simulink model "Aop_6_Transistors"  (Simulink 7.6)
settings: Solver=ode15s  StartTime=0.0  StopTime=10.0  RelTol=1e-3
libraries: fl_lib x20, elec_lib x8, nesl_utility x3

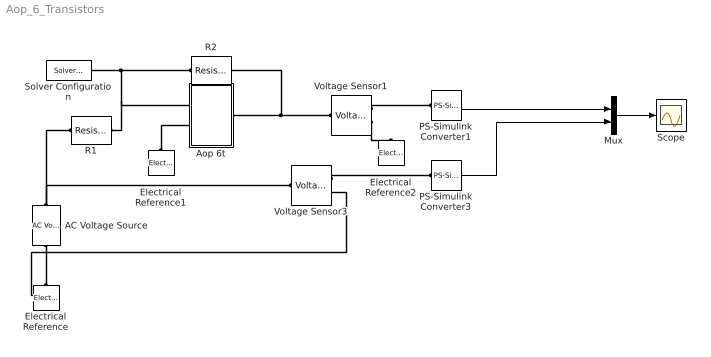
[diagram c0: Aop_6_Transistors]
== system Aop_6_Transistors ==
  AC Voltage Source : fl_lib/Electrical/Electrical Sources/AC Voltage Source  DialogController=NetworkEngine.DynNeDlgSource  SystemSampleTime=-1  amp=1 V  shift=0 rad  omega=1 Hz  i_Log=off  v_Log=off  LocalVarNames=|current|voltage|power  LocalVarDescs=|Current (A)|Voltage (V)|Power (W)  LocalVarLogging=[0 0 0]
  Aop 6t : Subsystem
  Electrical Reference : fl_lib/Electrical/Electrical Elements/Electrical Reference  DialogController=NetworkEngine.DynNeDlgSource  SystemSampleTime=-1  i_Log=off  LocalVarNames=|i  LocalVarDescs=|i  LocalVarLogging=[]
  Electrical Reference1 : fl_lib/Electrical/Electrical Elements/Electrical Reference  DialogController=NetworkEngine.DynNeDlgSource  SystemSampleTime=-1  i_Log=off  LocalVarNames=|i  LocalVarDescs=|i  LocalVarLogging=[]
  Electrical Reference2 : fl_lib/Electrical/Electrical Elements/Electrical Reference  DialogController=NetworkEngine.DynNeDlgSource  SystemSampleTime=-1  i_Log=off  LocalVarNames=|i  LocalVarDescs=|i  LocalVarLogging=[]
  Mux : Mux  Inputs=2
  PS-Simulink Converter1 : nesl_utility/PS-Simulink Converter  DialogController=NetworkEngine.DynNeUtilDlgSource  SystemSampleTime=-1  PhysicalDomain=network_engine_domain  LeftPortType=input  RightPortType=output  SubClassName=ps_output  Unit=1  AffineConversion=off
  PS-Simulink Converter3 : nesl_utility/PS-Simulink Converter  DialogController=NetworkEngine.DynNeUtilDlgSource  SystemSampleTime=-1  PhysicalDomain=network_engine_domain  LeftPortType=input  RightPortType=output  SubClassName=ps_output  Unit=1  AffineConversion=off
  R1 : fl_lib/Electrical/Electrical Elements/Resistor  DialogController=NetworkEngine.DynNeDlgSource  SystemSampleTime=-1  R=5 kOhm  i_Log=off  v_Log=off  LocalVarNames=|current|voltage|power  LocalVarDescs=|Resistor current (A)|Voltage across resistor (V)|Power (W)  LocalVarLogging=[0 0 0]
  R2 : fl_lib/Electrical/Electrical Elements/Resistor  DialogController=NetworkEngine.DynNeDlgSource  SystemSampleTime=-1  R=10 kOhm  i_Log=off  v_Log=off  LocalVarNames=|current|voltage|power  LocalVarDescs=|Resistor current (A)|Voltage across resistor (V)|Power (W)  LocalVarLogging=[0 0 0]
  Scope : Scope
  Solver Configuration : nesl_utility/Solver Configuration  DialogController=NetworkEngine.DynNeUtilDlgSource  SystemSampleTime=-1  PhysicalDomain=network_engine_domain  LeftPortType=input  RightPortType=generic  SubClassName=solver  Accelerate=off  Profile=off  ResidualTolerance=1e-9  MaxNonlinIter=12  MaxModeIter=2  DoFixedCost=off  UseLocalSampling=off  DoDC=off  LinearAlgebra=Sparse  LocalSolverSampleTime=.001  LocalSolverChoice=NE_BACKWARD_EULER_ADVANCER  UseLocalSolver=off
  Voltage Sensor1 : fl_lib/Electrical/Electrical Sensors/Voltage Sensor  DialogController=NetworkEngine.DynNeDlgSource  SystemSampleTime=-1  i1_Log=off  v1_Log=off  LocalVarNames=|i1|v1  LocalVarDescs=|i1|v1  LocalVarLogging=[]
  Voltage Sensor3 : fl_lib/Electrical/Electrical Sensors/Voltage Sensor  DialogController=NetworkEngine.DynNeDlgSource  SystemSampleTime=-1  i1_Log=off  v1_Log=off  LocalVarNames=|i1|v1  LocalVarDescs=|i1|v1  LocalVarLogging=[]
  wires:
  PS-Simulink Converter1/1 -> Mux/1
  Mux/1 -> Scope/1
  PS-Simulink Converter3/1 -> Mux/2
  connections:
  Electrical Reference/LConn1 -- Voltage Sensor3/RConn2 -- AC Voltage Source/RConn1
  AC Voltage Source/LConn1 -- Voltage Sensor3/LConn1 -- R1/LConn1
  Aop 6t/RConn1 -- R2/RConn1 -- Voltage Sensor1/LConn1
  R1/RConn1 -- Solver Configuration/RConn1 -- R2/LConn1 -- Aop 6t/LConn1
  Voltage Sensor3/RConn1 -- PS-Simulink Converter3/LConn1
  Voltage Sensor1/RConn2 -- Electrical Reference2/LConn1
  Voltage Sensor1/RConn1 -- PS-Simulink Converter1/LConn1
  Electrical Reference1/LConn1 -- Aop 6t/LConn2

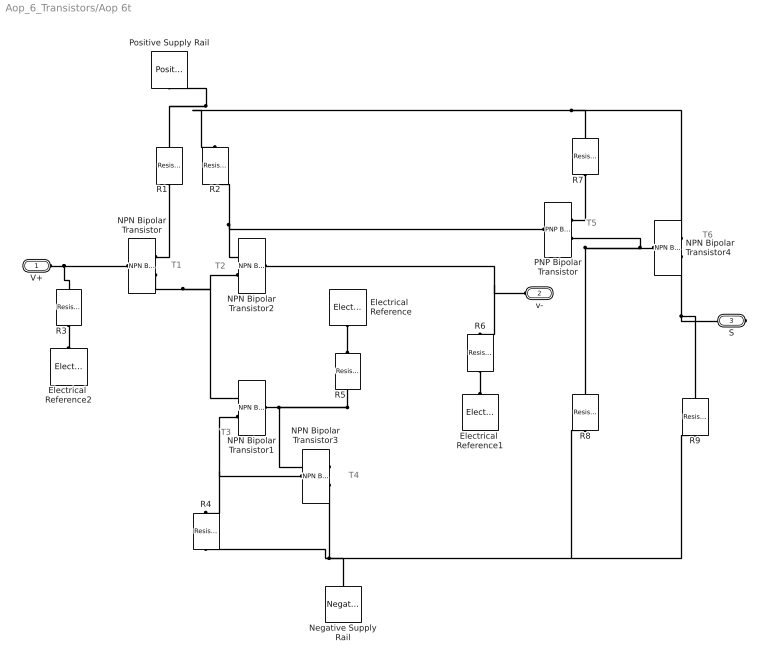
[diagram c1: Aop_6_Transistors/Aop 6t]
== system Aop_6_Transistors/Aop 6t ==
  note: T1
  note: T2
  note: T3
  note: T4
  note: T5
  note: T6
  Electrical  Reference : fl_lib/Electrical/Electrical Elements/Electrical Reference  DialogController=NetworkEngine.DynNeDlgSource  SystemSampleTime=-1  i_Log=off  LocalVarNames=|i  LocalVarDescs=|i  LocalVarLogging=0
  Electrical  Reference1 : fl_lib/Electrical/Electrical Elements/Electrical Reference  DialogController=NetworkEngine.DynNeDlgSource  SystemSampleTime=-1  i_Log=off  LocalVarNames=|i  LocalVarDescs=|i  LocalVarLogging=0
  Electrical  Reference2 : fl_lib/Electrical/Electrical Elements/Electrical Reference  DialogController=NetworkEngine.DynNeDlgSource  SystemSampleTime=-1  i_Log=off  LocalVarNames=|i  LocalVarDescs=|i  LocalVarLogging=0
  NPN Bipolar Transistor{,1..4} (5 alike) : elec_lib/Semiconductor Devices/NPN Bipolar Transistor  DialogController=NetworkEngine.DynNeDlgSource  SystemSampleTime=-1  parameterization=1  BF=100  IS=1e-14 A  VAF=200 V  hfe=100  hoe=5e-5 1/Ohm  Ic_h=1 mA  V1=0.55 V  I1=0.5 mA  BR=1  Tmeas=25 C  RC=0.01 Ohm  RE=1e-4 Ohm  RB=1 Ohm  C_BC=5 pF  C_BE=5 pF  TF=0 us  TR=0 us  LocalVarLogging=[]
  Negative Supply Rail : elec_lib/Sources/Negative Supply Rail  DialogController=NetworkEngine.DynNeDlgSource  SystemSampleTime=-1  v0=-15 V  current_Log=off  voltage_Log=off  power_Log=off  LocalVarNames=|current|voltage|power  LocalVarDescs=|Current (A)|Voltage (V)|Power (W)  LocalVarLogging=[0 0 0]
  PNP Bipolar Transistor : elec_lib/Semiconductor Devices/PNP Bipolar Transistor  DialogController=NetworkEngine.DynNeDlgSource  SystemSampleTime=-1  parameterization=1  BF=100  IS=1e-14 A  VAF=200 V  hfe=100  hoe=5e-5 1/Ohm  Ic_h=1 mA  V1=0.55 V  I1=0.5 mA  BR=1  Tmeas=25 C  RC=0.01 Ohm  RE=1e-4 Ohm  RB=1 Ohm  C_BC=5 pF  C_BE=5 pF  TF=0 us  TR=0 us  LocalVarLogging=[]
  Positive Supply Rail : elec_lib/Sources/Positive Supply Rail  DialogController=NetworkEngine.DynNeDlgSource  SystemSampleTime=-1  v0=15 V  current_Log=off  voltage_Log=off  power_Log=off  LocalVarNames=|current|voltage|power  LocalVarDescs=|Current (A)|Voltage (V)|Power (W)  LocalVarLogging=[0 0 0]
  R{1..3,6} (4 alike) : fl_lib/Electrical/Electrical Elements/Resistor  DialogController=NetworkEngine.DynNeDlgSource  SystemSampleTime=-1  R=4700 Ohm  i_Log=off  v_Log=off  LocalVarNames=|i|v  LocalVarDescs=|i|v  LocalVarLogging=[0 0]
  R4 : fl_lib/Electrical/Electrical Elements/Resistor  DialogController=NetworkEngine.DynNeDlgSource  SystemSampleTime=-1  R=1200 Ohm  i_Log=off  v_Log=off  LocalVarNames=|i|v  LocalVarDescs=|i|v  LocalVarLogging=[0 0]
  R5 : fl_lib/Electrical/Electrical Elements/Resistor  DialogController=NetworkEngine.DynNeDlgSource  SystemSampleTime=-1  R=27 kOhm  i_Log=off  v_Log=off  LocalVarNames=|i|v  LocalVarDescs=|i|v  LocalVarLogging=[0 0]
  R7 : fl_lib/Electrical/Electrical Elements/Resistor  DialogController=NetworkEngine.DynNeDlgSource  SystemSampleTime=-1  R=1 kOhm  i_Log=off  v_Log=off  LocalVarNames=|i|v  LocalVarDescs=|i|v  LocalVarLogging=[0 0]
  R8 : fl_lib/Electrical/Electrical Elements/Resistor  DialogController=NetworkEngine.DynNeDlgSource  SystemSampleTime=-1  R=24 kOhm  i_Log=off  v_Log=off  LocalVarNames=|i|v  LocalVarDescs=|i|v  LocalVarLogging=[0 0]
  R9 : fl_lib/Electrical/Electrical Elements/Resistor  DialogController=NetworkEngine.DynNeDlgSource  SystemSampleTime=-1  R=3 kOhm  i_Log=off  v_Log=off  LocalVarNames=|i|v  LocalVarDescs=|i|v  LocalVarLogging=[0 0]
  V+ : PMIOPort  Port=1  Side=Left
  v- : PMIOPort  Port=2  Side=Left
  S : PMIOPort  Port=3  Side=Right
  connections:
  Electrical  Reference/LConn1 -- R5/RConn1
  R6/LConn1 -- Electrical  Reference1/LConn1
  R3/LConn1 -- Electrical  Reference2/LConn1
  V+/RConn1 -- NPN Bipolar Transistor/LConn1 -- R3/RConn1
  R1/LConn1 -- NPN Bipolar Transistor/RConn1
  NPN Bipolar Transistor/RConn2 -- NPN Bipolar Transistor2/RConn2 -- NPN Bipolar Transistor1/RConn1
  NPN Bipolar Transistor1/LConn1 -- R5/LConn1 -- NPN Bipolar Transistor3/RConn1
  NPN Bipolar Transistor1/RConn2 -- R4/RConn1 -- NPN Bipolar Transistor3/LConn1
  v-/RConn1 -- R6/RConn1 -- NPN Bipolar Transistor2/LConn1
  PNP Bipolar Transistor/LConn1 -- R2/LConn1 -- NPN Bipolar Transistor2/RConn1
  NPN Bipolar Transistor3/RConn2 -- Negative Supply Rail/LConn1 -- R4/LConn1 -- R8/LConn1 -- R9/LConn1
  R7/LConn1 -- PNP Bipolar Transistor/RConn1
  NPN Bipolar Transistor4/LConn1 -- R8/RConn1 -- PNP Bipolar Transistor/RConn2
  NPN Bipolar Transistor4/RConn1 -- R7/RConn1 -- R1/RConn1 -- Positive Supply Rail/RConn1 -- R2/RConn1
  NPN Bipolar Transistor4/RConn2 -- R9/RConn1 -- S/RConn1
